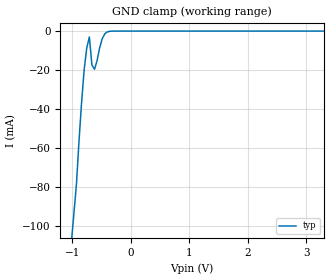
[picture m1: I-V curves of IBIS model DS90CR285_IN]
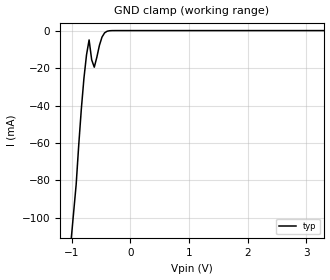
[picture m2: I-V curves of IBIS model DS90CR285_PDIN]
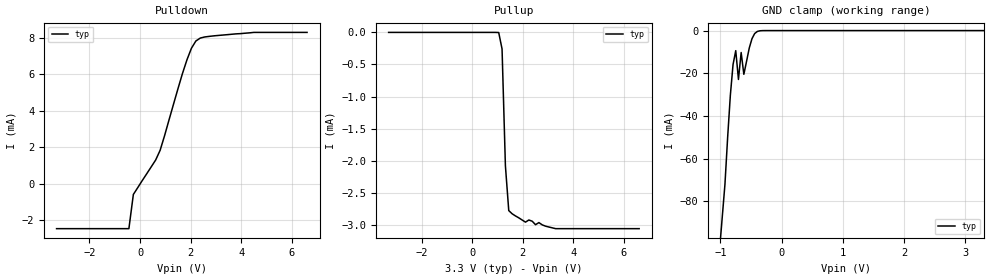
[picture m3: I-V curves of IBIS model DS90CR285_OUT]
|   National Semiconductor Corporation
|   Interface Products Group
|   Channel Link LVDS Transmitter
|   56L TSSOP
[IBIS Ver]   2.1
[Comment char]  |_char
[File name]   90cr285.ibs
[File Rev]   1.1
[Date]   2/19/98
[Source]   File originated at National Semiconductor Corporation.
   Interface Group/Analog Division. All data based on
   Empirical Measurements(Bench).
[Notes]   File created by SBH.
Rev. 1.1:
- changed Vref and Vmeas in OUT model to 1.2V
- modified by TSC on 10/31/02
[Disclaimer]
(C) Copyright National Semiconductor Corporation 1994
   All rights reserved
   National Semiconductor Corporation hereby grants
the user of this IBIS model a non-exclusive, nontransferable
license to use this IBIS model under the following terms.
Before using this IBIS model, the user should read this
license.  If the user does not accept these terms,  the
IBIS model should be returned to National within 30 days.
   The user is granted this license only to use the
IBIS model and is not granted rights to sell, load, rent,
lease or license the IBIS model in whole or in part, or in
modified form to anyone other than user. User may modify
the IBIS model to suit its specific applications but rights
to derivative works and such modifications shall belong to
National.
   This IBIS model is provided on an "AS IS" basis and
National makes absolutely no warranty with respect to the
information contained herein.NATIONAL DISCLAIMS AND CUSTOMER
WAIVES ALL WARRANTIES, EXPRESS OR IMPLIED, INCLUDING
WARRANTIES OF MERCHANTABILITY OR FITNESS FOR A PARTICULAR
PURPOSE. The entire risk as to quality and performance is
with the Customer. ACCORDINGLY, IN NO EVENT SHALL THE
COMPANY BE LIABLE FOR ANY DAMAGES, WHETHER IN CONTRACT OR
TORT,INCLUDING ANY LOST PROFITS OR OTHER INCIDENTAL,
CONSEQUENTIAL, EXEMPLARY, OR PUNITIVE DAMAGES ARISING OUT
OF THE USE OR APPLICATION OF THE IBIS model provided in
this package.Further, National reserves the right to make
changes without notice to any product herein to improve
reliability, function, or design. National does not convey
any license under patent rights or any other intellectual
property rights, including those of third parties.
   National is not obligated to provide maintenance or support
for the licensed IBIS model.
Contact National at ATTN:INTERFACE APPLICATIONS/IBIS MODELS.
2900 Semiconductor Drive, M/S A2595, Santa Clara, CA 95052-8090
[Copyright]   Copyright 1994, National Semiconductor, All Rights Reserved
[Component]   DS90CR285MTD
[Manufacturer]  National Semiconductor Corp
[Package]
|   typ   min   max
R_pkg   35.0m   NA   NA
L_pkg   4.31nH   NA   NA
C_pkg   0.70pF   NA   NA
[Pin]   signal_name   model_name   R_pin   L_pin   C_pin
1   VCC   POWER   50.0m   2.07n   0.429p
2   TxIN5   DS90CR285_IN   50.0m   1.49n   0.306p
3   TxIN6   DS90CR285_IN   50.0m   0.95n   0.146p
4   TxIN7   DS90CR285_IN   50.0m   0.95n   0.152p
5   GND   GND   50.0m   0.95n   0.152p
6   TxIN8   DS90CR285_IN   50.0m   0.95n   0.146p
7   TxIN9   DS90CR285_IN   50.0m   1.49n   0.306p
8   TxIN10   DS90CR285_IN   50.0m   2.07n   0.429p
9   Vcc   POWER   50.0m   2.07n   0.429p
10   TxIN11   DS90CR285_IN   50.0m   1.49n   0.306p
11   TxIN12   DS90CR285_IN   50.0m   0.95n   0.146p
12   TxIN13   DS90CR285_IN   50.0m   0.95n   0.152p
13   GND   GND   50.0m   0.95n   0.152p
14   TxIN14   DS90CR285_IN   50.0m   0.95n   0.146p
15   TxIN15   DS90CR285_IN   50.0m   1.49n   0.306p
16   TxIN16   DS90CR285_IN   50.0m   2.07n   0.429p
17   Vcc   POWER   50.0m   2.07n   0.429p
18   TxIN17   DS90CR285_IN   50.0m   1.49n   0.306p
19   TxIN18   DS90CR285_IN   50.0m   0.95n   0.146p
20   TxIN19   DS90CR285_IN   50.0m   0.95n   0.152p
21   GND   GND   50.0m   0.95n   0.152p
22   TxIN20   DS90CR285_IN   50.0m   0.95n   0.146p
23   TxIN21   DS90CR285_IN   50.0m   1.49n   0.306p
24   TxIN22   DS90CR285_IN   50.0m   2.07n   0.429p
25   TxIN23   DS90CR285_IN   50.0m   2.07n   0.429p
26   Vcc   POWER   50.0m   1.49n   0.306p
27   TxIN24   DS90CR285_IN   50.0m   0.95n   0.146p
28   TxIN25   DS90CR285_IN   50.0m   0.95n   0.152p
29   GND   GND   50.0m   0.95n   0.152p
30   TxIN26   DS90CR285_IN   50.0m   0.95n   0.146p
31   TxCLKIN   DS90CR285_IN   50.0m   1.49n   0.306p
32   PWRDWN*   DS90CR285_PDIN   50.0m   2.07n   0.429p
33   PLLGND   GND   50.0m   2.07n   0.429p
34   PLLVCC   POWER   50.0m   1.49n   0.306p
35   PLLGND   GND   50.0m   0.95n   0.146p
36   LVDSGND   GND   50.0m   0.95n   0.152p
37   TxOUT3+   DS90CR285_OUT   50.0m   0.95n   0.152p
38   TxOUT3-   DS90CR285_OUT   50.0m   0.95n   0.146p
39   TxCLKOUT+   DS90CR285_OUT   50.0m   1.49n   0.306p
40   TxCLKOUT-   DS90CR285_OUT   50.0m   2.07n   0.429p
41   TxOUT2+   DS90CR285_OUT   50.0m   2.07n   0.429p
42   TxOUT2-   DS90CR285_OUT   50.0m   1.49n   0.306p
43   LVDSGND   GND   50.0m   0.95n   0.146p
44   LVDSVCC   POWER   50.0m   0.95n   0.152p
45   TxOUT1+   DS90CR285_OUT   50.0m   0.95n   0.152p
46   TxOUT1-   DS90CR285_OUT   50.0m   0.95n   0.146p
47   TxOUT0+   DS90CR285_OUT   50.0m   1.49n   0.306p
48   TxOUT0-   DS90CR285_OUT   50.0m   2.07n   0.429p
49   LVDSGND   GND   50.0m   2.07n   0.429p
50   TxIN27   DS90CR285_IN   50.0m   2.07n   0.429p
51   TxIN0   DS90CR285_IN   50.0m   1.49n   0.306p
52   TxIN1   DS90CR285_IN   50.0m   0.95n   0.146p
53   GND   GND   50.0m   0.95n   0.152p
54   TxIN2   DS90CR285_IN   50.0m   0.95n   0.152p
55   TxIN3   DS90CR285_IN   50.0m   0.95n   0.146p
56   TxIN4   DS90CR285_IN   50.0m   1.49n   0.306p
[Diff_pin]   inv_pin   vdiff   tdelay_typ   tdelay_min   tdelay_max
| The '+' pin is Diff_pin and the '-' pin is the inv_pin
37   38   NA   0 0 0
39   40   NA   0 0 0
41   42   NA   0 0 0
45   46   NA   0 0 0
47   48   NA   0 0 0
| Models and submodels in the file (3): DS90CR285_IN (Input), DS90CR285_PDIN (Input), DS90CR285_OUT (3-state)
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|   Driver Input  MODEL
[Model]   DS90CR285_IN
Model_type   Input
|Signals   TxIN0 ~ TxIN20
Vinh = 2.0
Vinl = 0.8
|   typ   min   max
C_comp   5.863pF   NA   NA
|   typ   min   max
[Temperature Range]   25.0   NA   NA
[Voltage range]   3.3V   3.0V   3.6V
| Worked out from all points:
|   GND clamp passes 1 mA (typ) near -0.42 V on its own axis
[Power_clamp]
| Note that the[POWER_clamp]voltage table is referenced to Vcc
| and is calculated using Vtable=Vcc - Vmeasured.
|Voltage   I(typ)   I(min)   I(max)
-3V       0A         NA         NA
3V        0A         NA         NA
[GND_clamp]
|Voltage   I(typ)   I(min)   I(max)
-3.3V     -900mA     NA         NA
-926.5mV  -78.66mA   NA         NA
-838.2mV  -36.45mA   NA         NA
-794.1mV  -19.65mA   NA         NA
-750mV    -8.6mA     NA         NA
-705.9mV  -3.041mA   NA         NA
-661.8mV  -17.51mA   NA         NA
-617.7mV  -19.61mA   NA         NA
-485.3mV  -3.848mA   NA         NA
-441.2mV  -1.385mA   NA         NA
-352.9mV  -89.46uA   NA         NA
3.3V      0A         NA         NA
|   Driver PWRDWN* Input  MODEL
[Model]   DS90CR285_PDIN
Model_type   Input
|Signals   PWRDWN*
Vinh = 2.0
Vinl = 0.8
|   typ   min   max
C_comp   5.863pF   NA   NA
|   typ   min   max
[Temperature Range]   25.0   NA   NA
[Voltage range]   3.3V   3.0V   3.6V
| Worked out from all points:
|   GND clamp passes 1 mA (typ) near -0.43 V on its own axis
[Power_clamp]
| Note that the[POWER_clamp]voltage table is referenced to Vcc
| and is calculated using Vtable=Vcc - Vmeasured.
|Voltage   I(typ)   I(min)   I(max)
-3V       0A         NA         NA
3V        0A         NA         NA
[GND_clamp]
|Voltage   I(typ)   I(min)   I(max)
-3.3V     -900mA     NA         NA
-926.5mV  -82.06mA   NA         NA
-838.2mV  -41.78mA   NA         NA
-794.1mV  -25.51mA   NA         NA
-750mV    -12.98mA   NA         NA
-705.9mV  -4.994mA   NA         NA
-661.8mV  -15.62mA   NA         NA
-617.7mV  -19.54mA   NA         NA
-485.3mV  -3.454mA   NA         NA
-441.2mV  -1.208mA   NA         NA
-352.9mV  -73.7uA    NA         NA
3.3V      0A         NA         NA
|   Driver Output  MODEL
[Model]   DS90CR285_OUT
Model_type   3-state
| Signals   TxOUT0 ~ TxOUT2; TxCLKOUT
Vmeas = 1.2V   |This is 0.0v differential on ouput
Cref = 5pF   |Timing specification test load capacitance value
Rref = 100   |Note: 100 Ohm between the two driver outputs
Vref = 1.2   |Timing specification test load voltage; GND
| variable   typ   min   max
C_comp   6.763pF   NA   NA
|   typ   min   max
[Temperature Range]   25.0   NA   NA
[Voltage range]   3.3V   3.0V   3.6V
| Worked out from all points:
|   slope of the pulldown table from 0 to 0.495 V, typ, clamps not added: 469 ohm
|   GND clamp passes 1 mA (typ) near -0.42 V on its own axis
[Pulldown]
| Voltage   I(typ)   I(min)   I(max)
-3.3V     -2.453mA   NA         NA
-441.2mV  -2.453mA   NA         NA
-264.7mV  -577.4uA   NA         NA
617.6mV   1.312mA    NA         NA
794.1mV   1.846mA    NA         NA
1.676V    6.053mA    NA         NA
1.853V    6.801mA    NA         NA
2.029V    7.433mA    NA         NA
2.206V    7.835mA    NA         NA
2.559V    8.056mA    NA         NA
4.5V      8.306mA    NA         NA
6.6V      8.306mA    NA         NA
[Pullup]
| Note that the[Pullup]voltage table is referenced to Vcc
| and is calculated using Vtable=Vcc - Vmeasured.
|Voltage   I(typ)   I(min)   I(max)
-3.3V     4.294nA    NA         NA
1.05V     -1.983uA   NA         NA
1.182V    -257.7uA   NA         NA
1.315V    -2.078mA   NA         NA
1.447V    -2.776mA   NA         NA
2.109V    -2.956mA   NA         NA
2.241V    -2.923mA   NA         NA
2.506V    -2.996mA   NA         NA
2.638V    -2.963mA   NA         NA
2.903V    -3.019mA   NA         NA
3.3V      -3.058mA   NA         NA
6.6V      -3.058mA   NA         NA
[GND_clamp]
| Outputs in Tri-state.
| Voltage   I(typ)   I(min)   I(max)
-3.3V     -900mA     NA         NA
-926.5mV  -72mA      NA         NA
-838.2mV  -30.31mA   NA         NA
-794.1mV  -15.88mA   NA         NA
-750mV    -9.402mA   NA         NA
-705.9mV  -22.89mA   NA         NA
-661.8mV  -10.27mA   NA         NA
-617.7mV  -20.48mA   NA         NA
-529.4mV  -8.176mA   NA         NA
-485.3mV  -3.823mA   NA         NA
-397.1mV  -395.7uA   NA         NA
3.3V      0A         NA         NA
[POWER_clamp]
| Note that the[POWER_clamp]voltage table is referenced to Vcc
| and is calculated using Vtable=Vcc - Vmeasured.
| Outputs in Tri-state.
|Voltage   I(typ)   I(min)   I(max)
-3V       0A         NA         NA
3V        0A         NA         NA
[Ramp]
| Note: Ramp rate measured on single-ended Driver Output.
|   typ   min   max
dV/dt_r   135.0m/0.484n   NA   NA
dV/dt_f   135.0m/0.679n   NA   NA
R_load = 100Ohm | Note: This 100 Ohm is across the two driver output
